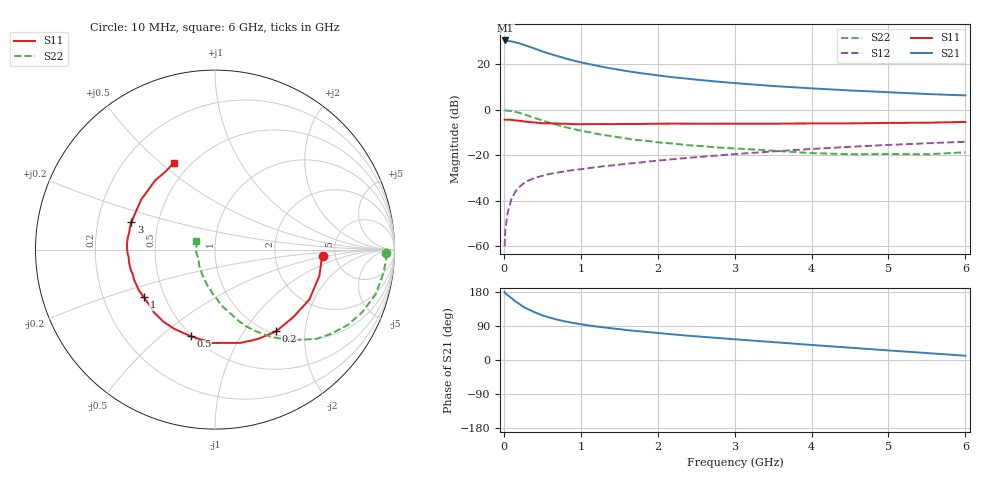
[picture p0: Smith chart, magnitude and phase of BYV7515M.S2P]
! SIEMENS Small Signal Semiconductors
! BFY420
! Si NPN RF SIEGET Grounded Emitter Transistor in MICRO-X
! VCE = 0.75 V  IC = 15 mA
! Common Emitter S-Parameters:  October  1996
# GHz  S  MA  R  50
!  f  S11  S21  S12  S22
! GHz  MAG  ANG  MAG  ANG  MAG  ANG  MAG  ANG
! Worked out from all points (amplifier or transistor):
!   36 points, 10 MHz to 6 GHz, reference 50 ohm
!   highest |S21| = 30.4 dB at 20 MHz (marker M1)
!   |S21| within 3 dB of that: start of sweep to 352.7 MHz
!   unconditionally stable (mu >= 1): 1.979 GHz to end of sweep
!   at 250 MHz: K = 0.26, MSG = 30.6 dB, |S12| = -32.6 dB
!   at 1.4 GHz: K = 0.89, MSG = 21.3 dB, |S12| = -24.6 dB
!   at 6 GHz: K = 1.11, MAG = 8.2 dB, |S12| = -14.2 dB
!   S11 on the Smith chart (normalised r, x): 10 MHz: 3.96, -0.47; 200 MHz: 1.05, -1.42; 500 MHz: 0.49, -0.63; 1 GHz: 0.38, -0.26; 3 GHz: 0.35, +0.14; 6 GHz: 0.41, +0.56
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0.01  0.6018 -3.6  32.96 178.9  0.001 93.3  0.9518 -1.2
0.02  0.5961 -6.1  32.98 176.0  0.0023 90.4  0.9548 -2.8
0.1  0.5947 -27.9  31.38 163.3  0.011 78.1  0.9286 -15.7
0.15  0.5765 -40.5  29.97 154.6  0.0159 72.4  0.8903 -23.2
0.2  0.5688 -53.2  28.57 148.0  0.0197 69.2  0.85 -29.7
0.25  0.5527 -64.3  26.82 141.0  0.0235 64.0  0.7983 -36.0
0.3  0.5391 -74.5  25.1 135.3  0.0266 61.3  0.7524 -41.4
0.4  0.5204 -91.6  21.88 126.1  0.0316 56.4  0.6568 -50.3
0.5  0.5015 -105.7  18.93 117.8  0.0351 53.6  0.5775 -57.3
0.6  0.4966 -117.4  16.75 111.7  0.0388 51.2  0.5116 -63.1
0.7  0.4938 -125.8  14.92 106.2  0.0414 49.7  0.4588 -68.2
0.8  0.488 -134.1  13.29 101.8  0.0443 48.9  0.4119 -72.3
1  0.4772 -146.2  10.93 94.5  0.0489 48.6  0.3451 -78.8
1.1  0.4806 -151.6  10.07 91.3  0.0517 48.6  0.3202 -82.4
1.4  0.4781 -163.1  7.952 83.6  0.0591 49.0  0.2612 -90.4
1.6  0.4832 -169.7  6.998 78.9  0.0646 48.5  0.2306 -95.7
2.2  0.4915 176.3  5.13 67.6  0.0813 47.4  0.1791 -108.8
3  0.4898 161.9  3.822 54.6  0.1052 44.0  0.1404 -124.2
3.5  0.4894 153.5  3.293 47.3  0.1204 40.9  0.1251 -134.6
4.5  0.4983 138.6  2.631 32.5  0.1521 32.7  0.1046 -155.6
5.5  0.5149 122.2  2.196 18.3  0.1821 23.2  0.1043 170.5
6  0.5357 115.1  2.048 11.3  0.1961 18.2  0.1156 155.5
